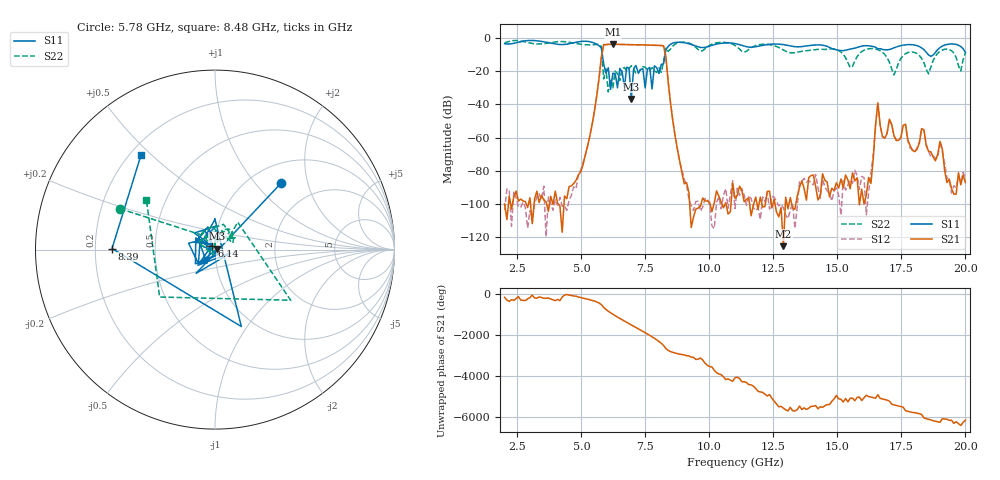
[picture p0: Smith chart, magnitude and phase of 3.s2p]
!Keysight Technologies,N5234A,MY52241180,A.10.60.03
!Date: Friday, January 20, 2023 09:33:15
!Correction: S11(Full 2 Port(1,2))
!S21(Full 2 Port(1,2))
!S12(Full 2 Port(1,2))
!S22(Full 2 Port(1,2))
!S2P File: Measurements: S11, S21, S12, S22:
# Hz S  dB  R 50
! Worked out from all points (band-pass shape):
!   201 points, 2 GHz to 20 GHz, reference 50 ohm
!   highest |S21| = -3.54 dB at 6.23 GHz (marker M1); lowest = -125.8 dB at 12.89 GHz (marker M2)
!   |S21| within 3 dB of the highest: 5.837 GHz to 8.238 GHz (2.401 GHz wide, 34.1 % of centre)
!   lowest |S11| = -36.7 dB at 6.95 GHz (marker M3), VSWR 1.03, Z = 51.4 + j0.548 ohm
!   |S11| at or under -10 dB: 5.82 GHz to 8.267 GHz (2.447 GHz wide, 34.7 % of centre); 18.56 GHz to 18.75 GHz (181.7 MHz wide, 0.974 % of centre)
!   |S22| runs from -32.4 to -1.3 dB; largest |S21 - S12| = 0.00021
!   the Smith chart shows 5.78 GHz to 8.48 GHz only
!   S11 on the Smith chart (normalised r, x): 5.78 GHz: 1.36, +1.38; 6.14 GHz: 0.96, +0.04; 8.39 GHz: 0.27, +0.00; 8.48 GHz: 0.24, +0.46
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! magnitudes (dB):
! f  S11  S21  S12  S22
! 2 GHz  -3.3  -100.2  -104.0  -2.7
! 5.06 GHz  -1.7  -76.8  -75.4  -3.7
! 5.78 GHz  -5.7  -11.3  -11.3  -4.8
! 5.87 GHz  -15.4  -3.7  -3.7  -24.5
! 6.14 GHz  -30.8  -3.6  -3.6  -24.7
! 6.23 GHz  -21.1  -3.5  -3.5  -29.9
! 6.86 GHz  -18.0  -3.7  -3.7  -18.1
! 6.95 GHz  -36.7  -3.8  -3.8  -16.6
! 7.13 GHz  -16.4  -3.9  -3.9  -21.5
! 7.49 GHz  -30.0  -4.0  -4.0  -17.4
! 8.03 GHz  -21.2  -4.2  -4.2  -17.7
! 8.39 GHz  -4.8  -26.2  -26.2  -7.8
! 8.48 GHz  -3.5  -38.9  -38.9  -6.5
! 8.93 GHz  -2.4  -81.5  -79.7  -2.3
! 11 GHz  -3.1  -96.8  -102.9  -4.2
! 12.89 GHz  -3.7  -125.8  -102.6  -7.0
! 14.06 GHz  -4.0  -82.7  -88.7  -6.9
! 16.31 GHz  -4.7  -87.8  -81.3  -6.2
! 16.58 GHz  -6.3  -39.0  -39.0  -6.8
! 16.76 GHz  -6.6  -59.3  -59.6  -8.4
! 17.03 GHz  -6.7  -48.9  -49.0  -14.4
! 20 GHz  -8.5  -87.3  -84.4  -8.8
